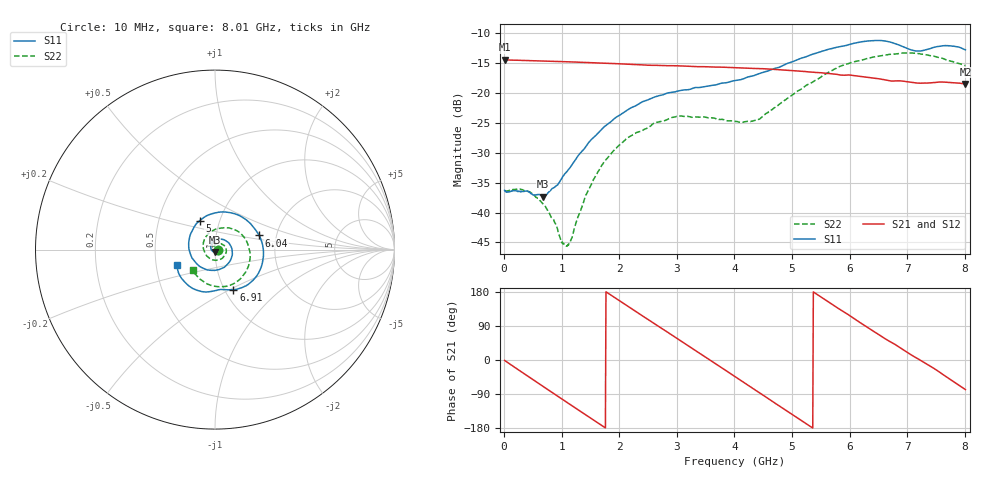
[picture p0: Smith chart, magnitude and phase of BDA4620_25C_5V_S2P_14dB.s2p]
!Agilent Technologies,E5071B,MY42404982,A.09.10
!Date: Wed May 06 09:01:09 2026
!Data & Calibration Information:
!Freq	S11:SOLT2(ON)	S21:SOLT2(ON)	S12:SOLT2(ON)	S22:SOLT2(ON)
# Hz S RI R 50
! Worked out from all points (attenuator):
!   801 points, 10 MHz to 8.01 GHz, reference 50 ohm
!   highest |S21| = -14.42 dB at 10 MHz (marker M1); lowest = -18.5 dB at 8.01 GHz (marker M2)
!   lowest |S11| = -37.4 dB at 680 MHz (marker M3), VSWR 1.03, Z = 49.7 - j1.32 ohm
!   |S11| at or under -10 dB: start of sweep to end of sweep
!   |S22| runs from -45.6 to -13.3 dB; largest |S21 - S12| = 0.00082
!   S11 on the Smith chart (normalised r, x): 10 MHz: 1.03, -0.00; 5 GHz: 0.80, +0.27; 6.04 GHz: 1.62, +0.27; 6.91 GHz: 1.10, -0.52; 8.01 GHz: 0.64, -0.12
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1e7  0.0153 -0.00108  0.19 -0.00398  0.1902 -0.00413  0.0152 -0.000658
4.2e8  0.00867 -0.0122  0.1359 -0.1285  0.1361 -0.1288  0.0134 -0.00666
6.8e8  -0.00275 -0.0133  0.0636 -0.1742  0.0637 -0.1745  0.00763 -0.00888
1.08e9  -0.0217 0.00153  -0.0642 -0.1712  -0.0644 -0.1714  -0.00427 -0.00302
1.16e9  -0.0231 0.00759  -0.0874 -0.1599  -0.0878 -0.1601  -0.00588 -0.000179
1.35e9  -0.0233 0.0226  -0.1342 -0.1211  -0.1344 -0.1214  -0.00795 0.00767
1.59e9  -0.013 0.042  -0.1702 -0.0551  -0.1705 -0.0552  -0.00574 0.0194
1.9e9  0.0159 0.058  -0.1719 0.0404  -0.1722 0.0405  0.00672 0.0322
2.68e9  0.0946 0.0023  0.00274 0.1704  0.00291 0.1706  0.0543 0.0177
3.4e9  0.0381 -0.1046  0.1587 0.0499  0.159 0.0498  0.0453 -0.0437
4.01e9  -0.0901 -0.0897  0.1179 -0.113  0.1181 -0.1133  -0.0231 -0.0534
4.42e9  -0.1448 0.00236  0.0141 -0.1595  0.014 -0.1597  -0.0595 -0.00945
5e9  -0.0857 0.1608  -0.124 -0.0918  -0.1242 -0.0919  -0.0359 0.089
5.35e9  0.0262 0.2091  -0.1494 -0.00395  -0.1497 -0.00397  0.0299 0.1191
5.65e9  0.1375 0.1888  -0.1282 0.0695  -0.1283 0.0696  0.0962 0.1155
6.04e9  0.2458 0.079  -0.0549 0.1296  -0.055 0.1298  0.1729 0.0525
6.37e9  0.2657 -0.0665  0.0228 0.1322  0.023 0.1322  0.1954 -0.0291
6.68e9  0.1901 -0.1904  0.0808 0.0977  0.0812 0.098  0.1779 -0.1119
6.91e9  0.1021 -0.224  0.1103 0.0608  0.1106 0.0611  0.1406 -0.1641
7.19e9  0.0278 -0.2226  0.1209 0.00591  0.1212 0.00605  0.0662 -0.2039
7.57e9  -0.0912 -0.2292  0.1037 -0.0676  0.1039 -0.0676  -0.0388 -0.1933
8.01e9  -0.2121 -0.088  0.0249 -0.1163  0.0252 -0.1166  -0.1239 -0.1151
